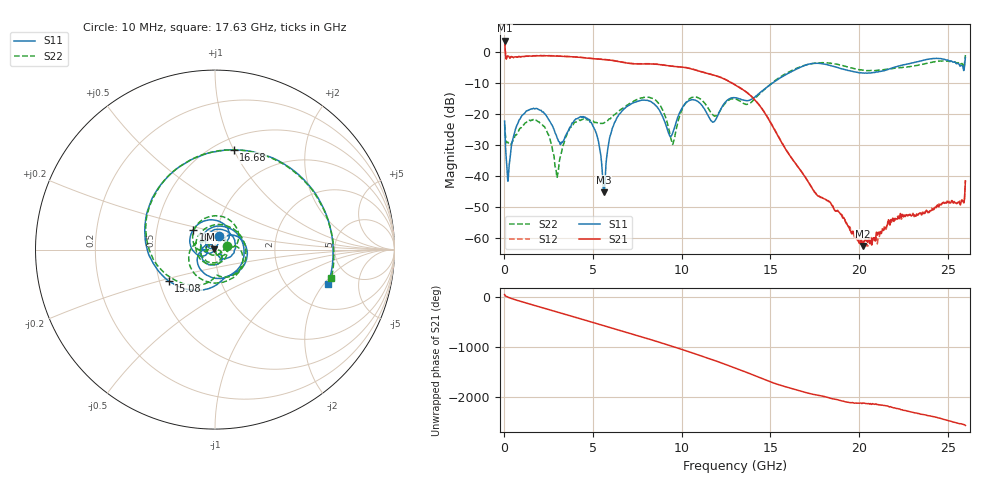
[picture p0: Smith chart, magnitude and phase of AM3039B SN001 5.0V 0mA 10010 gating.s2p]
!Agilent Technologies,E8364B,MY43040894,A.07.50.67
!Agilent E8364B: A.07.50.67
!Date: Tuesday, June 28, 2016 08:07:46
!Correction: S11(Full 2 Port(1,2))
!S21(Full 2 Port(1,2))
!S12(Full 2 Port(1,2))
!S22(Full 2 Port(1,2))
!S2P File: Measurements: S11, S21, S12, S22:
# Hz S  dB  R 50
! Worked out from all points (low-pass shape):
!   1601 points, 10 MHz to 26 GHz, reference 50 ohm
!   highest |S21| = 3.69 dB at 10 MHz (marker M1); lowest = -62.6 dB at 20.2 GHz (marker M2)
!   |S21| within 3 dB of the highest: start of sweep to 44.1 MHz
!   lowest |S11| = -45.3 dB at 5.598 GHz (marker M3), VSWR 1.01, Z = 49.5 + j0.185 ohm
!   |S11| at or under -10 dB: start of sweep to 15.12 GHz
!   |S22| runs from -40.6 to -1.0 dB; largest |S21 - S12| = 0.025
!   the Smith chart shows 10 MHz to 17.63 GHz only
!   S11 on the Smith chart (normalised r, x): 10 MHz: 1.03, +0.15; 10.41 GHz: 0.77, +0.17; 15.08 GHz: 0.56, -0.22; 16.68 GHz: 0.61, +1.00; 17.63 GHz: 3.28, -2.22
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1e7  -22.26 72.9  3.69 40.8  3.75 41.6  -23.35 16.0
7.24725e8  -23.44 141.0  -1.67 -74.3  -1.61 -74.2  -26.23 175.2
1.683106e9  -18.30 44.0  -1.24 -173.8  -1.20 -173.6  -21.81 43.0
2.722706e9  -23.99 -53.2  -1.26 80.2  -1.20 80.4  -32.04 -73.9
3.51865e9  -26.16 -41.9  -1.45 -0.8  -1.39 -0.6  -26.72 -32.6
4.347081e9  -20.99 -117.8  -1.76 -86.3  -1.72 -86.1  -21.83 -143.7
5.59785e9  -45.28 160.0  -2.38 144.3  -2.33 144.5  -22.95 -20.9
6.962325e9  -17.41 75.2  -3.60 1.9  -3.55 2.2  -17.02 81.5
8.684162e9  -18.27 -143.0  -4.00 179.9  -3.93 -179.8  -16.44 -166.1
1.0406e10  -15.69 138.0  -5.24 -14.5  -5.18 -14.3  -15.20 122.6
1.17055e10  -22.41 39.4  -7.28 -168.6  -7.23 -168.4  -19.91 8.2
1.3005e10  -14.71 -25.8  -10.61 25.0  -10.55 25.2  -15.11 -52.2
1.50842e10  -10.14 -145.8  -23.53 98.4  -23.39 98.8  -10.03 -157.5
1.667609e10  -4.95 79.4  -37.94 -70.7  -37.95 -70.1  -4.78 72.6
1.734208e10  -3.71 13.2  -43.78 -133.3  -44.03 -132.3  -3.72 12.9
1.763447e10  -3.62 -16.8  -46.18 -152.4  -46.19 -151.3  -3.51 -13.8
2.020098e10  -6.77 122.8  -62.59 46.4  -62.29 39.5  -5.80 133.5
2.167916e10  -5.49 21.5  -54.16 -23.6  -55.15 -24.4  -5.49 28.8
2.318983e10  -3.21 -92.3  -53.00 -146.6  -52.53 -149.6  -4.39 -81.2
2.429441e10  -2.06 178.2  -50.06 131.4  -50.55 132.0  -3.07 -165.2
2.526903e10  -3.15 93.5  -48.19 35.3  -48.06 35.4  -3.19 112.6
2.6e10  -1.76 -15.8  -41.58 -35.8  -41.48 -35.6  -0.95 16.7
